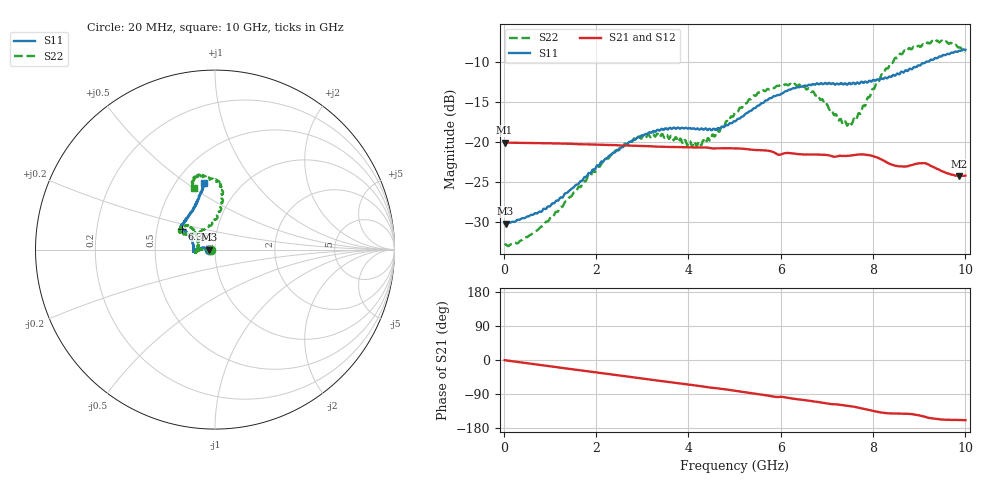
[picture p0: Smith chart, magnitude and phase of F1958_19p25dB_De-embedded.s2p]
! Integrated Device Technology
! Corporate Headquarters
! 6024 Silver Creek Valley Road
! San Jose, CA 95138  USA
! Phone:  1-408-284-8200
! Toll Free:  1-800-223-1366
! Webpage:  http://www.idt.com/
! Timing and RF Division
! 515 Groton Road, Suite 102
! Westford, MA 01886-6024
! Device:  F1958
! Description: 7-bit 0.25 dB Digital Step Attenuator
! Frequency:  0.001 -  6.000 GHz
! Package:  4x4 mm Thin QFN Plastic Package: 24 pin
! Ports:  2 RF, 12 DC
!  Pin  1  = D0
!  Pin  2  = VDD
!  Pin  3  = VMODE
!  Pin  4  = GND
!  Pin  5  = RF1  =  Port 1
!  Pin  6  = GND
!  Pin  7  = GND
!  Pin  8  = GND
!  Pin  9  = GND
!  Pin 10  = GND
!  Pin 11  = GND
!  Pin 12  = GND
!  Pin 13  = GND
!  Pin 14  = RF2  =  Port 2
!  Pin 15  = GND
!  Pin 16  = LE
!  Pin 17  = CLK
!  Pin 18  = DATA
!  Pin 19  = D6
!  Pin 20  = D5
!  Pin 21  = D4
!  Pin 22  = D3
!  Pin 23  = D2
!  Pin 24  = D1
! State:  77
! Atten State:  19.25 dB
! Voltage:  +3.30 Volts
! Current:  0.258 mA
! Data:  The device was measured on a F1958 evaluation board which has
!  individual transmission lines to the RF pins.  Data was collected
!  using a calibrated network analyzer.  The evaluation board was
!  de-embedded using Automatic Fixture Removal (AFR).
!  The reference plane is the edge of the package pin.
! Misc:
!  Action Tracker AT0419
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# GHz S dB R 50
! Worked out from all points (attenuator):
!   500 points, 20 MHz to 10 GHz, reference 50 ohm
!   highest |S21| = -20.11 dB at 20 MHz (marker M1); lowest = -24.3 dB at 9.86 GHz (marker M2)
!   lowest |S11| = -30.2 dB at 40 MHz (marker M3), VSWR 1.06, Z = 47 - j0.0412 ohm
!   |S11| at or under -10 dB: start of sweep to 9.158 GHz; 9.177467 GHz to 9.203354 GHz (25.89 MHz wide, 0.282 % of centre)
!   |S22| runs from -33.0 to -7.4 dB; largest |S21 - S12| = 0.00042
!   S11 on the Smith chart (normalised r, x): 20 MHz: 0.94, -0.00; 6.36 GHz: 0.67, +0.16; 10 GHz: 0.68, +0.58
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0.02  -30.19 -178.9  -20.11 -0.4  -20.10 -0.4  -32.90 -178.1
0.04  -30.21 -179.2  -20.11 -0.7  -20.11 -0.7  -32.81 -177.2
0.32  -29.74 175.1  -20.14 -5.4  -20.14 -5.4  -32.60 178.8
0.72  -28.97 172.6  -20.18 -12.0  -20.17 -11.9  -31.08 179.6
1.7  -24.87 171.1  -20.32 -27.8  -20.31 -27.8  -25.25 178.6
2.6  -20.59 177.0  -20.47 -42.3  -20.45 -42.3  -20.46 -177.4
3.36  -18.60 -175.6  -20.62 -54.7  -20.62 -54.8  -19.30 -170.3
4.24  -18.51 -179.1  -20.72 -68.6  -20.73 -68.7  -20.04 167.3
4.5  -18.58 175.1  -20.83 -73.2  -20.83 -73.2  -19.43 151.6
5.02  -17.44 160.6  -20.82 -81.3  -20.83 -81.3  -16.29 138.2
5.58  -15.20 150.4  -21.08 -91.1  -21.09 -91.1  -13.84 138.5
6  -14.07 148.2  -21.59 -97.1  -21.61 -97.1  -12.86 146.0
6.36  -13.19 147.9  -21.53 -103.6  -21.55 -103.5  -13.10 151.7
6.68  -12.86 146.4  -21.60 -108.5  -21.62 -108.4  -13.78 152.7
7.3  -12.68 140.7  -21.77 -118.5  -21.78 -118.4  -17.16 131.4
7.5  -12.72 138.1  -21.75 -121.8  -21.75 -121.7  -17.49 112.9
7.68  -12.68 135.2  -21.60 -125.5  -21.59 -125.5  -16.48 96.0
8.34  -11.89 119.0  -22.70 -140.8  -22.70 -140.9  -10.69 81.3
8.68  -11.24 112.3  -23.11 -141.7  -23.11 -141.7  -8.62 86.0
9.26  -9.75 104.7  -23.04 -153.7  -23.05 -153.7  -7.55 99.1
9.86  -8.68 99.8  -24.28 -158.1  -24.31 -158.1  -8.26 108.3
10  -8.54 99.8  -24.24 -158.8  -24.28 -158.8  -8.78 109.2
